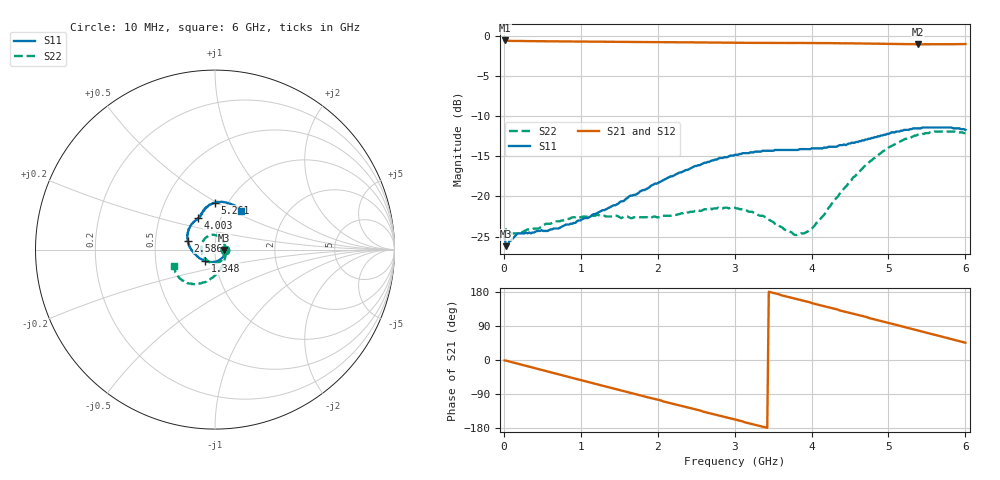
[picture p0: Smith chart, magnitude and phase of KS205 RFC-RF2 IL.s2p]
!Agilent	"Technologies,E5071B,JP1KK00126,A.08.11"
!Date:	Wed	Mar	27	12:07:20	2013
!Data	&	Calibration	Information:
!Freq	S11:SOLT2(ON)	S21:SOLT2(ON)	S12:SOLT2(ON)	S22:SOLT2(ON)
#	Hz	S	dB	R	50
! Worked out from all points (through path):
!   301 points, 10 MHz to 6 GHz, reference 50 ohm
!   highest |S21| = -0.54 dB at 10 MHz (marker M1); lowest = -1.0 dB at 5.381 GHz (marker M2)
!   group delay of S21, straight-line fit = 145 ps
!   lowest |S11| = -26.2 dB at 29.97 MHz (marker M3), VSWR 1.10, Z = 55.1 - j0.266 ohm
!   |S11| at or under -10 dB: start of sweep to end of sweep
!   |S22| runs from -25.1 to -11.9 dB; largest |S21 - S12| = 0.016
!   S11 on the Smith chart (normalised r, x): 10 MHz: 1.12, -0.01; 1.348 GHz: 0.89, -0.11; 2.586 GHz: 0.73, +0.07; 4.003 GHz: 0.78, +0.29; 5.261 GHz: 0.87, +0.49; 6 GHz: 1.19, +0.56
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1e7  -25.20 -2.9  -0.54 -1.1  -0.54 -1.1  -25.10 -2.3
2.996667e7  -26.20 -2.8  -0.57 -1.8  -0.57 -1.8  -24.10 -1.5
1.897e8  -24.60 -16.1  -0.60 -10.4  -0.60 -10.4  -24.60 -13.1
5.291333e8  -24.30 -52.1  -0.64 -28.3  -0.64 -28.3  -23.50 -41.2
1.0283e9  -22.80 -105.0  -0.68 -54.5  -0.68 -54.6  -22.50 -81.2
1.347767e9  -21.50 -132.0  -0.70 -71.2  -0.70 -71.2  -22.50 -106.0
1.667233e9  -19.90 -154.0  -0.73 -87.8  -0.73 -87.8  -22.70 -133.0
2.006667e9  -18.30 -173.0  -0.75 -105.0  -0.75 -105.0  -22.60 -166.0
2.326133e9  -16.90 173.0  -0.77 -122.0  -0.77 -122.0  -22.10 163.0
2.5857e9  -15.90 162.0  -0.79 -136.0  -0.79 -136.0  -21.70 139.0
3.005e9  -14.80 145.0  -0.83 -157.0  -0.83 -157.0  -21.40 104.0
3.504167e9  -14.30 129.0  -0.85 177.0  -0.85 177.0  -23.20 59.2
3.7837e9  -14.20 122.0  -0.86 162.0  -0.86 162.0  -24.80 18.2
4.003333e9  -14.00 118.0  -0.87 150.0  -0.87 150.0  -24.00 -21.1
4.0233e9  -14.00 118.0  -0.87 149.0  -0.87 149.0  -23.80 -24.5
4.5025e9  -13.40 110.0  -0.90 124.0  -0.90 124.0  -18.10 -80.5
4.7421e9  -12.80 106.0  -0.93 111.0  -0.93 111.0  -15.80 -97.6
5.001667e9  -12.20 98.7  -0.97 97.8  -0.97 97.8  -13.90 -112.0
5.261233e9  -11.70 90.0  -1.00 84.2  -1.00 84.3  -12.70 -124.0
5.381033e9  -11.50 85.2  -1.02 78.0  -1.02 78.1  -12.30 -130.0
5.680533e9  -11.40 72.0  -1.02 62.4  -1.02 62.5  -11.90 -143.0
6e9  -11.70 56.6  -0.99 45.6  -0.99 45.6  -12.10 -158.0
